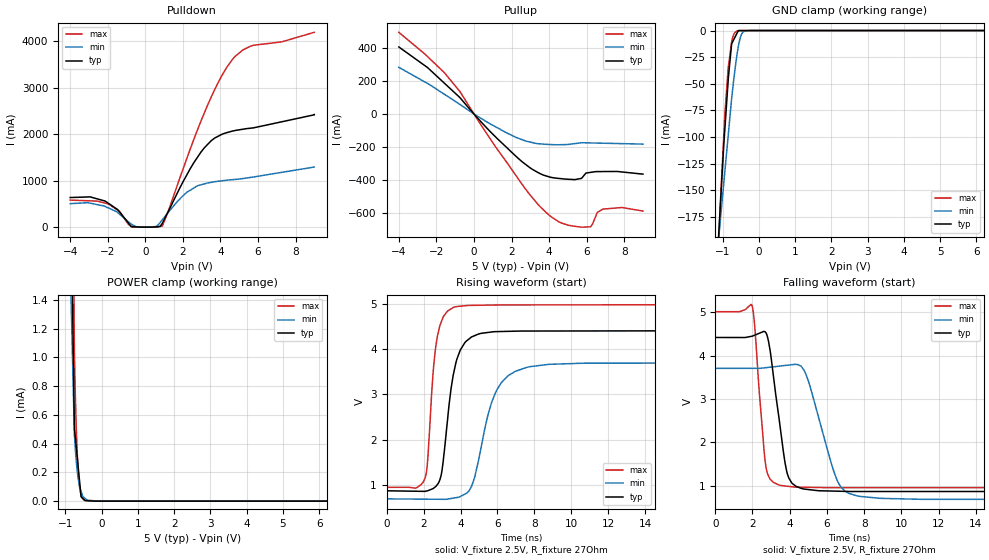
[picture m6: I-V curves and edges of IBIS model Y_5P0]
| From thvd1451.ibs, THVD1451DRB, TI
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|   Y_5P0 Model
[Model]   Y_5P0
Model_type   3-state
Polarity   Non-Inverting
Vmeas = 2.5
Vref = 2.5
Cref = 50pF
Rref = 27
|   typ   min   max
C_comp   28.949pF   27.267pF   29.083pF
|  Where Nom  PVT is Nominal Process,   3.3V,  25C
|   Fast PVT is Strong Process,   3.6V, -40C
|   Slow PVT is Weak Process,   3V, 150C
[Voltage Range]   5   4.5   5.5
|Junction Temperature
[Temperature Range]   25   150   -40
[Pullup Reference]   5   4.5   5.5
[Pulldown Reference]   0   -0   -0
[Power Clamp Reference]   5   4.5   5.5
[GND Clamp Reference]   0   0   0
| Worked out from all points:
|   slope of the pulldown table from 0 to 0.75 V, typ, clamps not added: 59.6 ohm
|   slope of the pullup table from 0 to 0.75 V, typ, clamps not added: 8.09 ohm
|   GND clamp passes 1 mA (typ) near -0.58 V on its own axis
|   falling waveform, V_fixture 2.5V, R_fixture 27Ohm: 20-80 % time 660ps typ, 1.19ns min, 430ps max; typ from 4.42 V to 0.865 V
|   rising waveform, V_fixture 2.5V, R_fixture 27Ohm: 20-80 % time 675ps typ, 1.13ns min, 450ps max; typ from 0.868 V to 4.41 V
[Pulldown]
|   Voltage   I(typ)   I(min)   I(max)
-4V       637.2mA    505.8mA    582.4mA
-2.145V   561.6mA    446.6mA    517.9mA
-1.365V   323.7mA    277.1mA    333.9mA
-749.3mV  12.12mA    63.54mA    10.68mA
575.9mV   6.935mA    14.46mA    1.908mA
908.7mV   84.92mA    161.2mA    24.38mA
1.945V    926.8mA    652.7mA    1.179A
2.959V    1.613A     910.7mA    2.279A
3.7V      1.918A     977.7mA    2.963A
4.628V    2.066A     1.021A     3.604A
5.749V    2.136A     1.079A     3.913A
9V        2.425A     1.294A     4.193A
[GND Clamp]
|   Voltage   I(typ)   I(min)   I(max)
-4V       -2.011A    -1.275A    -2.643A
-1.211V   -254.2mA   -233.1mA   -280.6mA
-1.05V    -157.8mA   -174.1mA   -155.3mA
-965.7mV  -107.4mA   -143.2mA   -98.96mA
-935.5mV  -92.21mA   -132.2mA   -78.72mA
-844.5mV  -46.72mA   -98.84mA   -35.24mA
-749.3mV  -12.43mA   -63.98mA   -10.82mA
-687.2mV  -8.274mA   -45.08mA   -3.498mA
-610.6mV  -3.136mA   -24.93mA   -588uA
-516.1mV  -62.98uA   -7.384mA   -54.95uA
-379.6mV  -36.24uA   -325.9uA   -40.17uA
9V        0A         0A         0A
[Pullup]
|   Voltage   I(typ)   I(min)   I(max)
-4V       404.6mA    281.6mA    493mA
-1.58V    186.4mA    119.4mA    249.8mA
-749.3mV  99.06mA    58.1mA     135.6mA
2.403V    -272.7mA   -148.4mA   -399.3mA
3.144V    -336.7mA   -173.7mA   -509.9mA
4.072V    -382.1mA   -184.6mA   -617.5mA
5.369V    -396.5mA   -179.1mA   -678.4mA
6.214V    -352.8mA   -175mA     -681.6mA
6.572V    -347.9mA   -175.9mA   -594.6mA
6.867V    -347.8mA   -176.6mA   -574.7mA
7.892V    -350.4mA   -179.2mA   -565mA
9V        -363.3mA   -182mA     -586.4mA
[POWER Clamp]
|   Voltage   I(typ)   I(min)   I(max)
-4V       245.5mA    143.2mA    363.8mA
-1.072V   6.093mA    3.783mA    10.75mA
-749.3mV  510.3uA    466.7uA    1.062mA
-724.9mV  446.9uA    367.9uA    758.6uA
-697.6mV  375.8uA    279.9uA    511.9uA
-671.6mV  308.1uA    212.3uA    337.7uA
-641.8mV  230.4uA    151.2uA    201.3uA
-614.5mV  159.3uA    110.2uA    120.4uA
-565mV    30.41uA    68.41uA    44.12uA
-453.2mV  3.518uA    19.27uA    6.168uA
-1.267mV  0A         0A         0A
9V        0A         0A         0A
[Ramp]
R_load = 27
|   typ   min   max
dV/dt_r   2.12741/6.73639e-10   1.8087/1.12807e-09   2.4264/4.48476e-10
dV/dt_f   2.13457/6.56035e-10   1.81471/1.18432e-09   2.43961/4.30181e-10
[Falling Waveform]
V_fixture = 2.5V
V_fixture_min = 2.25V
V_fixture_max = 2.75V
R_fixture = 27Ohm
C_fixture = 0F
|   Time   V(typ)   V(min)   V(max)
0s        4.423V     3.709V     5.018V
1.98ns    4.452V     3.71V      5.153V
2.711ns   4.537V     3.725V     1.464V
3.408ns   2.611V     3.759V     1.018V
3.835ns   1.338V     3.78V      988.5mV
4.148ns   1.047V     3.795V     972.9mV
4.872ns   917mV      3.571V     962.8mV
6.598ns   872.1mV    1.08V      955mV
7.595ns   865.2mV    766.9mV    954.9mV
30ns      865mV      684.4mV    952.1mV
[Rising Waveform]
V_fixture = 2.5V
V_fixture_min = 2.25V
V_fixture_max = 2.75V
R_fixture = 27Ohm
C_fixture = 0F
|   Time   V(typ)   V(min)   V(max)
0s        867.6mV    688.8mV    944.1mV
2.07ns    854.9mV    682.3mV    1.139V
2.198ns   865.8mV    681.9mV    1.432V
2.724ns   995.6mV    680.2mV    4.231V
2.997ns   1.32V      679.4mV    4.644V
3.61ns    3.437V     705.6mV    4.923V
4.598ns   4.271V     965.4mV    4.969V
5.969ns   4.389V     3.102V     4.977V
7.595ns   4.401V     3.598V     4.979V
30ns      4.413V     3.703V     4.988V
